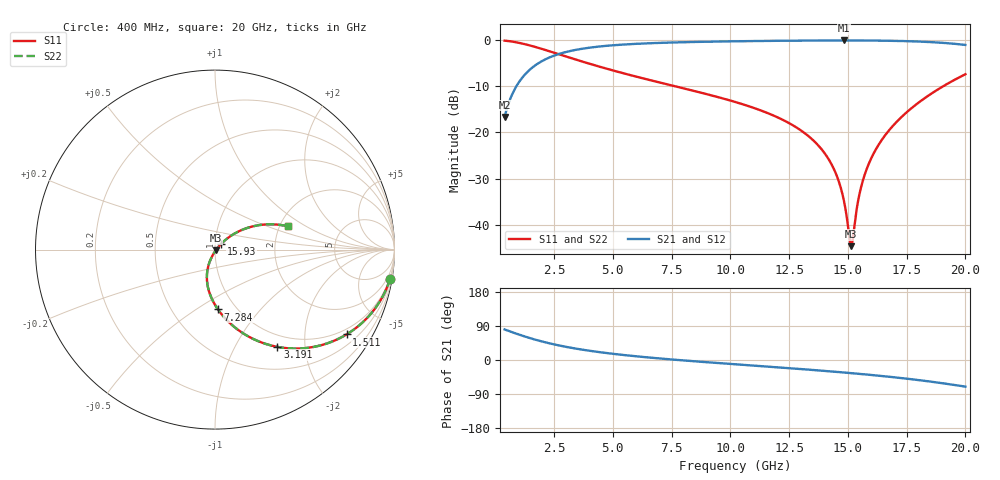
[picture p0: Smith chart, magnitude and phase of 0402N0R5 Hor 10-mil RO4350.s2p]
# GHz S MA R 50
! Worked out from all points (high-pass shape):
!   1960 points, 400 MHz to 20 GHz, reference 50 ohm
!   highest |S21| = -0.06 dB at 14.83 GHz (marker M1); lowest = -16.7 dB at 400 MHz (marker M2)
!   |S21| within 3 dB of the highest: 2.67 GHz to end of sweep
!   lowest |S11| = -44.7 dB at 15.15 GHz (marker M3), VSWR 1.01, Z = 50.5 - j0.321 ohm
!   |S11| at or under -10 dB: 7.663 GHz to 19.05 GHz (11.39 GHz wide, 85.3 % of centre)
!   |S22| runs from -44.7 to -0.1 dB; largest |S21 - S12| = 0
!   S11 on the Smith chart (normalised r, x): 400 MHz: 1, -12; 1.511 GHz: 0.81, -3.21; 3.191 GHz: 0.81, -1.51; 7.284 GHz: 0.82, -0.62; 15.93 GHz: 1.07, +0.07; 20 GHz: 2.22, +0.70
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0.4  0.9891 -9.4  0.1468 80.6  0.1468 80.6  0.9891 -9.4
0.880245  0.9505 -20.1  0.3103 69.8  0.3103 69.8  0.9505 -20.1
1.510567  0.8722 -32.8  0.4887 57.2  0.4887 57.2  0.8722 -32.8
3.191424  0.6442 -57.3  0.7638 32.6  0.7638 32.6  0.6442 -57.3
3.671669  0.5902 -62.3  0.806 27.6  0.806 27.6  0.5902 -62.3
5.112404  0.4622 -74.2  0.8851 15.6  0.8851 15.6  0.4622 -74.2
6.943338  0.3506 -85.4  0.9344 4.3  0.9344 4.3  0.3506 -85.4
7.283512  0.3339 -87.1  0.9404 2.5  0.9404 2.5  0.3339 -87.1
10.205  0.2142 -100.5  0.9735 -11.3  0.9735 -11.3  0.2142 -100.5
12.156  0.1401 -108.5  0.9859 -20.0  0.9859 -20.0  0.1401 -108.5
13.46667  0.08493 -113.1  0.9914 -26.1  0.9914 -26.1  0.08493 -113.1
14.3171  0.04462 -113.7  0.9933 -30.3  0.9933 -30.3  0.04462 -113.7
14.60725  0.02988 -111.5  0.9936 -31.8  0.9936 -31.8  0.02988 -111.5
14.82736  0.01849 -105.5  0.9937 -32.9  0.9937 -32.9  0.01849 -105.5
15.06748  0.007233 -71.3  0.9936 -34.2  0.9936 -34.2  0.007233 -71.3
15.14752  0.005853 -32.9  0.9935 -34.7  0.9935 -34.7  0.005853 -32.9
15.21756  0.007258 0.3  0.9934 -35.1  0.9934 -35.1  0.007258 0.3
15.52772  0.0234 37.8  0.9929 -36.8  0.9929 -36.8  0.0234 37.8
15.92792  0.04814 42.9  0.9915 -39.1  0.9915 -39.1  0.04814 42.9
16.73834  0.1044 41.7  0.9861 -44.1  0.9861 -44.1  0.1044 41.7
18.11904  0.221 33.6  0.9644 -53.8  0.9644 -53.8  0.221 33.6
20  0.4274 17.7  0.8883 -70.3  0.8883 -70.3  0.4274 17.7
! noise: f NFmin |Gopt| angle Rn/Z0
0.4  0.001458  0.87  6.548  0.002407
2.571  0.004449  0.6571  11.7  0.002451
4.752  0.007126  0.6054  15.36  0.003281
6.933  0.009799  0.5847  19.38  0.004191
9.104  0.01268  0.5807  23.47  0.005293
11.29  0.01604  0.5893  27.55  0.006771
13.47  0.0202  0.6094  31.58  0.008913
15.64  0.02566  0.6403  35.55  0.01227
17.82  0.03349  0.6826  39.58  0.01818
20  0.0459  0.7367  43.72  0.03014
